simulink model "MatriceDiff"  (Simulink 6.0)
settings: Solver=ode45  StartTime=0  StopTime=17*t0  RelTol=1e-3
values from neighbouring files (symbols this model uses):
  b = S/Sm    (= 0.1)    [Constantes.m]    (also in ConstantesBck.m)
  beta = 0.95    [Constantes.m]    (also in ConstantesBck.m; ResCourV1.m = 1; ResCrV1.m = 1; ResEnerV1.m = 1)
  C = 1    [Constantes.m]    (also in ConstantesBck.m)
  gk = 36    [Constantes.m]    (also in ConstantesBck.m; sim_hh.m)
  gl = 0.3    [Constantes.m]    (also in ConstantesBck.m; sim_hh.m)
  gna = 120    [Constantes.m]    (also in ConstantesBck.m; sim_hh.m)
  h0 = 0.5961    [Constantes.m]    (also in ConstantesBck.m)
  m0 = 0.0529    [Constantes.m]    (also in ConstantesBck.m)
  mK = 0    [Constantes.m]    (also in ConstantesBck.m)
  mL = 0    [Constantes.m]    (also in ConstantesBck.m)
  mNa = 0    [Constantes.m]    (also in ConstantesBck.m)
  N = [6,8,5,5,7,1,2,6,9,1,1,9,4,8,8,7]    [Constantes.m]    (also in ConstantesBck.m; ImpedanceZtissus.m = 100; Ztissus.m = 100; charge.m = N(:,2))
  n0 = 0.3177    [Constantes.m]    (also in ConstantesBck.m)
  rapportIE = 10    [Constantes.m]
  Sm = 3.14e-2    (= 0.0314)    [Constantes.m]    (also in ConstantesBck.m = 0.000314)
  t0 = 2E-3    (= 0.002)    [Constantes.m]    (also in ConstantesBck.m = 0.001)
  Vk = -82    [Constantes.m]    (also in ConstantesBck.m)
  Vl = -59    [Constantes.m]    (also in ConstantesBck.m)
  Vna = 45    [Constantes.m]    (also in ConstantesBck.m)
  Vr = -70    [Constantes.m]    (also in ConstantesBck.m)
undefined symbols (not defined in the file or in its folder): ln
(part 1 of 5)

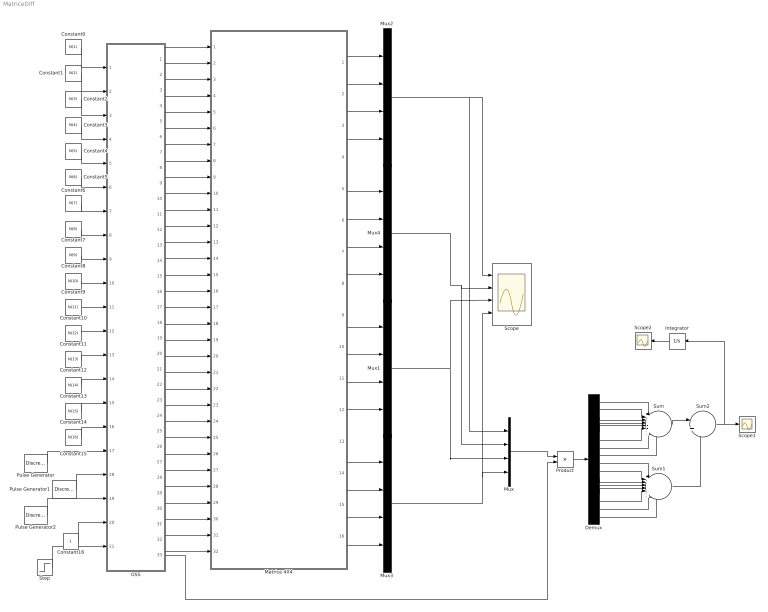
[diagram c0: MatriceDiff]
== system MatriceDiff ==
  Constant0 : Constant  Value=N(1)
  Constant1 : Constant  Value=N(2)
  Constant10 : Constant  Value=N(11)
  Constant11 : Constant  Value=N(12)
  Constant12 : Constant  Value=N(13)
  Constant13 : Constant  Value=N(14)
  Constant14 : Constant  Value=N(15)
  Constant15 : Constant  Value=N(16)
  Constant16 : Constant
  Constant2 : Constant  Value=N(3)
  Constant3 : Constant  Value=N(4)
  Constant4 : Constant  Value=N(5)
  Constant5 : Constant  Value=N(6)
  Constant6 : Constant  Value=N(7)
  Constant7 : Constant  Value=N(8)
  Constant8 : Constant  Value=N(9)
  Constant9 : Constant  Value=N(10)
  Demux : Demux  Outputs=16
  Integrator : Integrator  Orientation=left
  Matrice 4X4 : Subsystem
  Mux{,1..4} (5 alike) : Mux
  OSS : Stateflow chart
  Product : Product
  Pulse Generator : DiscretePulseGenerator  PulseType=Time based  Period=2*t0  PulseWidth=50  PhaseDelay=2*t0
  Pulse Generator1 : DiscretePulseGenerator  PulseType=Time based  Period=4*t0  PulseWidth=50  PhaseDelay=3*t0
  Pulse Generator2 : DiscretePulseGenerator  PulseType=Time based  Period=8*t0  PulseWidth=50  PhaseDelay=5*t0
  Scope : Scope  NumInputPorts=4
  Scope1 : Scope
  Scope2 : Scope
  Step : Step  Time=t0  SampleTime=0
  Sum : Sum  Inputs=|++++++++
  Sum1 : Sum  Inputs=|++++++++
  Sum2 : Sum  Inputs=|++
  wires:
  Matrice 4X4/13(Out12) -> Mux3/1
  Matrice 4X4/14(Out13) -> Mux3/2
  Matrice 4X4/15(Out14) -> Mux3/3
  Matrice 4X4/16(Out15) -> Mux3/4
  Constant14/1 -> OSS/15(u14)
  Constant13/1 -> OSS/14(u13)
  Constant12/1 -> OSS/13(u12)
  Constant11/1 -> OSS/12(u11)
  Constant10/1 -> OSS/11(u10)
  Constant9/1 -> OSS/10(u9)
  Constant8/1 -> OSS/9(u8)
  Constant7/1 -> OSS/8(u7)
  Constant6/1 -> OSS/7(u6)
  Constant5/1 -> OSS/6(u5)
  Constant4/1 -> OSS/5(u4)
  Constant3/1 -> OSS/4(u3)
  Constant2/1 -> OSS/3(u2)
  Constant1/1 -> OSS/2(u1)
  Constant0/1 -> OSS/1(u0)
  Constant15/1 -> OSS/16(u15)
  OSS/5(S2) -> Matrice 4X4/5(S2)
  OSS/6(Ref2) -> Matrice 4X4/6(Ref2)
  OSS/7(S3) -> Matrice 4X4/7(S3)
  OSS/8(Ref3) -> Matrice 4X4/8(Ref3)
  OSS/9(S4) -> Matrice 4X4/9(S4)
  OSS/10(Ref4) -> Matrice 4X4/10(Ref4)
  OSS/11(S5) -> Matrice 4X4/11(S5)
  OSS/12(Ref5) -> Matrice 4X4/12(Ref5)
  OSS/13(S6) -> Matrice 4X4/13(S6)
  OSS/14(Ref6) -> Matrice 4X4/14(Ref6)
  OSS/15(S7) -> Matrice 4X4/15(S7)
  OSS/16(Ref7) -> Matrice 4X4/16(Ref7)
  OSS/17(S8) -> Matrice 4X4/17(S8)
  OSS/18(Ref8) -> Matrice 4X4/18(Ref8)
  OSS/19(S9) -> Matrice 4X4/19(S9)
  OSS/20(Ref9) -> Matrice 4X4/20(Ref9)
  OSS/21(S10) -> Matrice 4X4/21(S10)
  OSS/22(Ref10) -> Matrice 4X4/22(Ref10)
  OSS/23(S11) -> Matrice 4X4/23(S11)
  OSS/24(Ref11) -> Matrice 4X4/24(Ref11)
  OSS/25(S12) -> Matrice 4X4/25(S12)
  OSS/26(Ref12) -> Matrice 4X4/26(Ref12)
  OSS/27(S13) -> Matrice 4X4/27(S13)
  OSS/28(Ref13) -> Matrice 4X4/28(Ref13)
  OSS/29(S14) -> Matrice 4X4/29(S14)
  OSS/30(Ref14) -> Matrice 4X4/30(Ref14)
  OSS/31(S15) -> Matrice 4X4/31(S15)
  OSS/32(Ref15) -> Matrice 4X4/32(Ref15)
  OSS/4(Ref1) -> Matrice 4X4/4(Ref1)
  OSS/3(S1) -> Matrice 4X4/3(S1)
  OSS/2(Ref0) -> Matrice 4X4/2(Ref0)
  OSS/1(S0) -> Matrice 4X4/1(S0)
  Pulse Generator/1 -> OSS/17(tc0)
  Pulse Generator2/1 -> OSS/19(tc2)
  Pulse Generator1/1 -> OSS/18(tc1)
  Mux3/1 -> Scope/4, Mux/4
  Matrice 4X4/9(Out8) -> Mux1/1
  Matrice 4X4/10(Out9) -> Mux1/2
  Matrice 4X4/12(Out11) -> Mux1/4
  Matrice 4X4/11(Out10) -> Mux1/3
  Matrice 4X4/5(Out4) -> Mux4/1
  Matrice 4X4/6(Out5) -> Mux4/2
  Matrice 4X4/7(Out6) -> Mux4/3
  Matrice 4X4/8(Out7) -> Mux4/4
  Matrice 4X4/1(Out0) -> Mux2/1
  Matrice 4X4/2(Out1) -> Mux2/2
  Matrice 4X4/4(Out3) -> Mux2/4
  Matrice 4X4/3(Out2) -> Mux2/3
  Mux1/1 -> Scope/3, Mux/3
  Mux4/1 -> Scope/2, Mux/2
  Mux2/1 -> Scope/1, Mux/1
  Constant16/1 -> OSS/20(dyn)
  OSS/33(MatCourant) -> Product/2
  Mux/1 -> Product/1
  Product/1 -> Demux/1
  Demux/1 -> Sum/1
  Demux/2 -> Sum/2
  Demux/3 -> Sum/3
  Demux/4 -> Sum/4
  Demux/5 -> Sum/5
  Demux/6 -> Sum/6
  Demux/7 -> Sum/7
  Demux/8 -> Sum/8
  Demux/9 -> Sum1/1
  Demux/10 -> Sum1/2
  Demux/11 -> Sum1/3
  Demux/12 -> Sum1/4
  Demux/13 -> Sum1/5
  Demux/14 -> Sum1/6
  Demux/15 -> Sum1/7
  Demux/16 -> Sum1/8
  Sum/1 -> Sum2/1
  Sum1/1 -> Sum2/2
  Sum2/1 -> Scope1/1, Integrator/1
  Integrator/1 -> Scope2/1
  Step/1 -> OSS/21(rst)

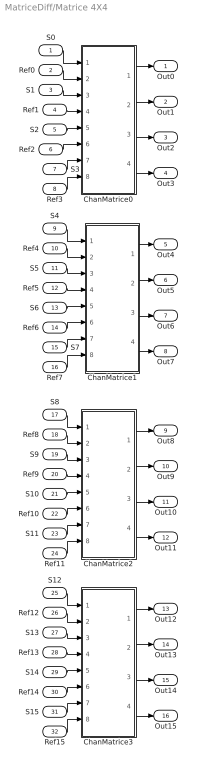
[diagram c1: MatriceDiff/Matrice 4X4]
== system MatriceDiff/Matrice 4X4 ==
  S0 : Inport  Port=1  LatchInput=off
  Ref0 : Inport  Port=2  LatchInput=off
  S1 : Inport  Port=3  LatchInput=off
  Ref1 : Inport  Port=4  LatchInput=off
  S2 : Inport  Port=5  LatchInput=off
  Ref2 : Inport  Port=6  LatchInput=off
  S3 : Inport  Port=7  LatchInput=off
  Ref3 : Inport  Port=8  LatchInput=off
  S4 : Inport  Port=9  LatchInput=off
  Ref4 : Inport  Port=10  LatchInput=off
  S5 : Inport  Port=11  LatchInput=off
  Ref5 : Inport  Port=12  LatchInput=off
  S6 : Inport  Port=13  LatchInput=off
  Ref6 : Inport  Port=14  LatchInput=off
  S7 : Inport  Port=15  LatchInput=off
  Ref7 : Inport  Port=16  LatchInput=off
  S8 : Inport  Port=17  LatchInput=off
  Ref8 : Inport  Port=18  LatchInput=off
  S9 : Inport  Port=19  LatchInput=off
  Ref9 : Inport  Port=20  LatchInput=off
  S10 : Inport  Port=21  LatchInput=off
  Ref10 : Inport  Port=22  LatchInput=off
  S11 : Inport  Port=23  LatchInput=off
  Ref11 : Inport  Port=24  LatchInput=off
  S12 : Inport  Port=25  LatchInput=off
  Ref12 : Inport  Port=26  LatchInput=off
  S13 : Inport  Port=27  LatchInput=off
  Ref13 : Inport  Port=28  LatchInput=off
  S14 : Inport  Port=29  LatchInput=off
  Ref14 : Inport  Port=30  LatchInput=off
  S15 : Inport  Port=31  LatchInput=off
  Ref15 : Inport  Port=32  LatchInput=off
  ChanMatrice0 : Subsystem
  ChanMatrice1 : Subsystem
  ChanMatrice2 : Subsystem
  ChanMatrice3 : Subsystem
  Out0 : Outport
  Out1 : Outport  Port=2
  Out2 : Outport  Port=3
  Out3 : Outport  Port=4
  Out4 : Outport  Port=5
  Out5 : Outport  Port=6
  Out6 : Outport  Port=7
  Out7 : Outport  Port=8
  Out8 : Outport  Port=9
  Out9 : Outport  Port=10
  Out10 : Outport  Port=11
  Out11 : Outport  Port=12
  Out12 : Outport  Port=13
  Out13 : Outport  Port=14
  Out14 : Outport  Port=15
  Out15 : Outport  Port=16
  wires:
  S0/1 -> ChanMatrice0/1(S0)
  ChanMatrice0/1(Out0) -> Out0/1
  Ref0/1 -> ChanMatrice0/2(Ref0)
  S1/1 -> ChanMatrice0/3(S1)
  ChanMatrice0/2(Out1) -> Out1/1
  ChanMatrice0/3(Out2) -> Out2/1
  ChanMatrice0/4(Out3) -> Out3/1
  ChanMatrice1/1(Out0) -> Out4/1
  ChanMatrice1/2(Out1) -> Out5/1
  ChanMatrice1/3(Out2) -> Out6/1
  ChanMatrice1/4(Out3) -> Out7/1
  ChanMatrice2/1(Out0) -> Out8/1
  ChanMatrice2/2(Out1) -> Out9/1
  ChanMatrice2/3(Out2) -> Out10/1
  ChanMatrice2/4(Out3) -> Out11/1
  ChanMatrice3/1(Out0) -> Out12/1
  ChanMatrice3/2(Out1) -> Out13/1
  ChanMatrice3/3(Out2) -> Out14/1
  ChanMatrice3/4(Out3) -> Out15/1
  S2/1 -> ChanMatrice0/5(S2)
  S3/1 -> ChanMatrice0/7(S3)
  S4/1 -> ChanMatrice1/1(S0)
  S5/1 -> ChanMatrice1/3(S1)
  S6/1 -> ChanMatrice1/5(S2)
  S7/1 -> ChanMatrice1/7(S3)
  S12/1 -> ChanMatrice3/1(S0)
  S13/1 -> ChanMatrice3/3(S1)
  S14/1 -> ChanMatrice3/5(S2)
  S15/1 -> ChanMatrice3/7(S3)
  S8/1 -> ChanMatrice2/1(S0)
  S9/1 -> ChanMatrice2/3(S1)
  S10/1 -> ChanMatrice2/5(S2)
  S11/1 -> ChanMatrice2/7(S3)
  Ref1/1 -> ChanMatrice0/4(Ref1)
  Ref2/1 -> ChanMatrice0/6(Ref2)
  Ref3/1 -> ChanMatrice0/8(Ref3)
  Ref4/1 -> ChanMatrice1/2(Ref0)
  Ref5/1 -> ChanMatrice1/4(Ref1)
  Ref6/1 -> ChanMatrice1/6(Ref2)
  Ref7/1 -> ChanMatrice1/8(Ref3)
  Ref8/1 -> ChanMatrice2/2(Ref0)
  Ref9/1 -> ChanMatrice2/4(Ref1)
  Ref10/1 -> ChanMatrice2/6(Ref2)
  Ref11/1 -> ChanMatrice2/8(Ref3)
  Ref12/1 -> ChanMatrice3/2(Ref0)
  Ref13/1 -> ChanMatrice3/4(Ref1)
  Ref14/1 -> ChanMatrice3/6(Ref2)
  Ref15/1 -> ChanMatrice3/8(Ref3)

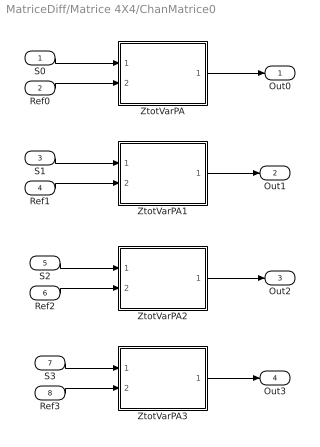
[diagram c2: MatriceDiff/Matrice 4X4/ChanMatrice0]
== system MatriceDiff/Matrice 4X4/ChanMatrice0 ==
  S0 : Inport  Port=1  LatchInput=off
  Ref0 : Inport  Port=2  LatchInput=off
  S1 : Inport  Port=3  LatchInput=off
  Ref1 : Inport  Port=4  LatchInput=off
  S2 : Inport  Port=5  LatchInput=off
  Ref2 : Inport  Port=6  LatchInput=off
  S3 : Inport  Port=7  LatchInput=off
  Ref3 : Inport  Port=8  LatchInput=off
  ZtotVarPA : Subsystem
  ZtotVarPA1 : Subsystem
  ZtotVarPA2 : Subsystem
  ZtotVarPA3 : Subsystem
  Out0 : Outport
  Out1 : Outport  Port=2
  Out2 : Outport  Port=3
  Out3 : Outport  Port=4
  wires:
  S0/1 -> ZtotVarPA/1(InZtot)
  Ref0/1 -> ZtotVarPA/2(InVref)
  ZtotVarPA/1(OutZtot) -> Out0/1
  ZtotVarPA1/1(OutZtot) -> Out1/1
  ZtotVarPA2/1(OutZtot) -> Out2/1
  ZtotVarPA3/1(OutZtot) -> Out3/1
  S1/1 -> ZtotVarPA1/1(InZtot)
  Ref1/1 -> ZtotVarPA1/2(InVref)
  S2/1 -> ZtotVarPA2/1(InZtot)
  Ref2/1 -> ZtotVarPA2/2(InVref)
  S3/1 -> ZtotVarPA3/1(InZtot)
  Ref3/1 -> ZtotVarPA3/2(InVref)

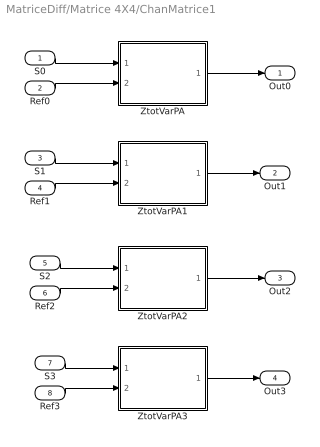
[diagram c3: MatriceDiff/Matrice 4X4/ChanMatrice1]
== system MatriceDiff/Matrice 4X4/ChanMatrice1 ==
  S0 : Inport  Port=1  LatchInput=off
  Ref0 : Inport  Port=2  LatchInput=off
  S1 : Inport  Port=3  LatchInput=off
  Ref1 : Inport  Port=4  LatchInput=off
  S2 : Inport  Port=5  LatchInput=off
  Ref2 : Inport  Port=6  LatchInput=off
  S3 : Inport  Port=7  LatchInput=off
  Ref3 : Inport  Port=8  LatchInput=off
  ZtotVarPA : Subsystem
  ZtotVarPA1 : Subsystem
  ZtotVarPA2 : Subsystem
  ZtotVarPA3 : Subsystem
  Out0 : Outport
  Out1 : Outport  Port=2
  Out2 : Outport  Port=3
  Out3 : Outport  Port=4
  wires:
  S0/1 -> ZtotVarPA/1(InZtot)
  Ref0/1 -> ZtotVarPA/2(InVref)
  ZtotVarPA/1(OutZtot) -> Out0/1
  ZtotVarPA1/1(OutZtot) -> Out1/1
  ZtotVarPA2/1(OutZtot) -> Out2/1
  ZtotVarPA3/1(OutZtot) -> Out3/1
  S1/1 -> ZtotVarPA1/1(InZtot)
  Ref1/1 -> ZtotVarPA1/2(InVref)
  S2/1 -> ZtotVarPA2/1(InZtot)
  Ref2/1 -> ZtotVarPA2/2(InVref)
  S3/1 -> ZtotVarPA3/1(InZtot)
  Ref3/1 -> ZtotVarPA3/2(InVref)

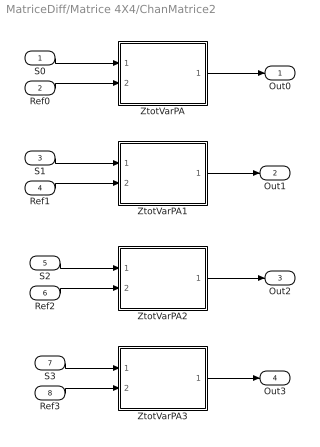
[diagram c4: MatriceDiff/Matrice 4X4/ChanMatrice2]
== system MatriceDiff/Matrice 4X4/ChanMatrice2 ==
  S0 : Inport  Port=1  LatchInput=off
  Ref0 : Inport  Port=2  LatchInput=off
  S1 : Inport  Port=3  LatchInput=off
  Ref1 : Inport  Port=4  LatchInput=off
  S2 : Inport  Port=5  LatchInput=off
  Ref2 : Inport  Port=6  LatchInput=off
  S3 : Inport  Port=7  LatchInput=off
  Ref3 : Inport  Port=8  LatchInput=off
  ZtotVarPA : Subsystem
  ZtotVarPA1 : Subsystem
  ZtotVarPA2 : Subsystem
  ZtotVarPA3 : Subsystem
  Out0 : Outport
  Out1 : Outport  Port=2
  Out2 : Outport  Port=3
  Out3 : Outport  Port=4
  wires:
  S0/1 -> ZtotVarPA/1(InZtot)
  Ref0/1 -> ZtotVarPA/2(InVref)
  ZtotVarPA/1(OutZtot) -> Out0/1
  ZtotVarPA1/1(OutZtot) -> Out1/1
  ZtotVarPA2/1(OutZtot) -> Out2/1
  ZtotVarPA3/1(OutZtot) -> Out3/1
  S1/1 -> ZtotVarPA1/1(InZtot)
  Ref1/1 -> ZtotVarPA1/2(InVref)
  S2/1 -> ZtotVarPA2/1(InZtot)
  Ref2/1 -> ZtotVarPA2/2(InVref)
  S3/1 -> ZtotVarPA3/1(InZtot)
  Ref3/1 -> ZtotVarPA3/2(InVref)

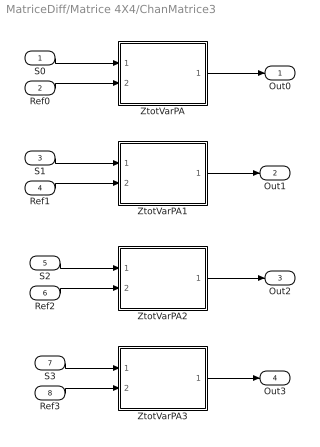
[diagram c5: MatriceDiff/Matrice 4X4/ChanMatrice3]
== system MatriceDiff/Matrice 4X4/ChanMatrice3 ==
  S0 : Inport  Port=1  LatchInput=off
  Ref0 : Inport  Port=2  LatchInput=off
  S1 : Inport  Port=3  LatchInput=off
  Ref1 : Inport  Port=4  LatchInput=off
  S2 : Inport  Port=5  LatchInput=off
  Ref2 : Inport  Port=6  LatchInput=off
  S3 : Inport  Port=7  LatchInput=off
  Ref3 : Inport  Port=8  LatchInput=off
  ZtotVarPA : Subsystem
  ZtotVarPA1 : Subsystem
  ZtotVarPA2 : Subsystem
  ZtotVarPA3 : Subsystem
  Out0 : Outport
  Out1 : Outport  Port=2
  Out2 : Outport  Port=3
  Out3 : Outport  Port=4
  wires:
  S0/1 -> ZtotVarPA/1(InZtot)
  Ref0/1 -> ZtotVarPA/2(InVref)
  ZtotVarPA/1(OutZtot) -> Out0/1
  ZtotVarPA1/1(OutZtot) -> Out1/1
  ZtotVarPA2/1(OutZtot) -> Out2/1
  ZtotVarPA3/1(OutZtot) -> Out3/1
  S1/1 -> ZtotVarPA1/1(InZtot)
  Ref1/1 -> ZtotVarPA1/2(InVref)
  S2/1 -> ZtotVarPA2/1(InZtot)
  Ref2/1 -> ZtotVarPA2/2(InVref)
  S3/1 -> ZtotVarPA3/1(InZtot)
  Ref3/1 -> ZtotVarPA3/2(InVref)

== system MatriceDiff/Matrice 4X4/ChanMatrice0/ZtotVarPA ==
  InZtot : Inport  Port=1  LatchInput=off
  InVref : Inport  Port=2  LatchInput=off
  Gain : Gain
  Sum : Sum  Inputs=|++
  ZTissusVar : Subsystem
  ZietVar : Subsystem
  OutZtot : Outport
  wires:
  ZietVar/1(OutZiet) -> Gain/1
  ZTissusVar/1(Vout) -> Sum/1
  InZtot/1 -> ZTissusVar/1(IStim), ZietVar/1(InZiet)
  Gain/1 -> Sum/2
  Sum/1 -> OutZtot/1
  InVref/1 -> ZTissusVar/2(Vref)

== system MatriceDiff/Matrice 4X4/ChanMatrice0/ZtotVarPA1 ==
  InZtot : Inport  Port=1  LatchInput=off
  InVref : Inport  Port=2  LatchInput=off
  Gain : Gain
  Sum : Sum  Inputs=|++
  ZTissusVar : Subsystem
  ZietVar : Subsystem
  OutZtot : Outport
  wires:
  ZietVar/1(OutZiet) -> Gain/1
  ZTissusVar/1(Vout) -> Sum/1
  InZtot/1 -> ZTissusVar/1(IStim), ZietVar/1(InZiet)
  Gain/1 -> Sum/2
  Sum/1 -> OutZtot/1
  InVref/1 -> ZTissusVar/2(Vref)

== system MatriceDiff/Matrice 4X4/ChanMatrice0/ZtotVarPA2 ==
  InZtot : Inport  Port=1  LatchInput=off
  InVref : Inport  Port=2  LatchInput=off
  Gain : Gain
  Sum : Sum  Inputs=|++
  ZTissusVar : Subsystem
  ZietVar : Subsystem
  OutZtot : Outport
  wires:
  ZietVar/1(OutZiet) -> Gain/1
  ZTissusVar/1(Vout) -> Sum/1
  InZtot/1 -> ZTissusVar/1(IStim), ZietVar/1(InZiet)
  Gain/1 -> Sum/2
  Sum/1 -> OutZtot/1
  InVref/1 -> ZTissusVar/2(Vref)

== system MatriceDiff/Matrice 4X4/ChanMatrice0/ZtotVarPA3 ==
  InZtot : Inport  Port=1  LatchInput=off
  InVref : Inport  Port=2  LatchInput=off
  Gain : Gain
  Sum : Sum  Inputs=|++
  ZTissusVar : Subsystem
  ZietVar : Subsystem
  OutZtot : Outport
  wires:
  ZietVar/1(OutZiet) -> Gain/1
  ZTissusVar/1(Vout) -> Sum/1
  InZtot/1 -> ZTissusVar/1(IStim), ZietVar/1(InZiet)
  Gain/1 -> Sum/2
  Sum/1 -> OutZtot/1
  InVref/1 -> ZTissusVar/2(Vref)

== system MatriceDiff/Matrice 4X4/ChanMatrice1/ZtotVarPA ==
  InZtot : Inport  Port=1  LatchInput=off
  InVref : Inport  Port=2  LatchInput=off
  Gain : Gain
  Sum : Sum  Inputs=|++
  ZTissusVar : Subsystem
  ZietVar : Subsystem
  OutZtot : Outport
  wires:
  ZietVar/1(OutZiet) -> Gain/1
  ZTissusVar/1(Vout) -> Sum/1
  InZtot/1 -> ZTissusVar/1(IStim), ZietVar/1(InZiet)
  Gain/1 -> Sum/2
  Sum/1 -> OutZtot/1
  InVref/1 -> ZTissusVar/2(Vref)

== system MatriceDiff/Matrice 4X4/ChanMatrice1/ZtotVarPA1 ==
  InZtot : Inport  Port=1  LatchInput=off
  InVref : Inport  Port=2  LatchInput=off
  Gain : Gain
  Sum : Sum  Inputs=|++
  ZTissusVar : Subsystem
  ZietVar : Subsystem
  OutZtot : Outport
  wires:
  ZietVar/1(OutZiet) -> Gain/1
  ZTissusVar/1(Vout) -> Sum/1
  InZtot/1 -> ZTissusVar/1(IStim), ZietVar/1(InZiet)
  Gain/1 -> Sum/2
  Sum/1 -> OutZtot/1
  InVref/1 -> ZTissusVar/2(Vref)

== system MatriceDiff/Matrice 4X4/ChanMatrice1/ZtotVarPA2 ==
  InZtot : Inport  Port=1  LatchInput=off
  InVref : Inport  Port=2  LatchInput=off
  Gain : Gain
  Sum : Sum  Inputs=|++
  ZTissusVar : Subsystem
  ZietVar : Subsystem
  OutZtot : Outport
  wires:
  ZietVar/1(OutZiet) -> Gain/1
  ZTissusVar/1(Vout) -> Sum/1
  InZtot/1 -> ZTissusVar/1(IStim), ZietVar/1(InZiet)
  Gain/1 -> Sum/2
  Sum/1 -> OutZtot/1
  InVref/1 -> ZTissusVar/2(Vref)

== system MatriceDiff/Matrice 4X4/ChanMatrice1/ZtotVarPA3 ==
  InZtot : Inport  Port=1  LatchInput=off
  InVref : Inport  Port=2  LatchInput=off
  Gain : Gain
  Sum : Sum  Inputs=|++
  ZTissusVar : Subsystem
  ZietVar : Subsystem
  OutZtot : Outport
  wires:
  ZietVar/1(OutZiet) -> Gain/1
  ZTissusVar/1(Vout) -> Sum/1
  InZtot/1 -> ZTissusVar/1(IStim), ZietVar/1(InZiet)
  Gain/1 -> Sum/2
  Sum/1 -> OutZtot/1
  InVref/1 -> ZTissusVar/2(Vref)

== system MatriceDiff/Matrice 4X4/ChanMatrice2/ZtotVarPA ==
  InZtot : Inport  Port=1  LatchInput=off
  InVref : Inport  Port=2  LatchInput=off
  Gain : Gain
  Sum : Sum  Inputs=|++
  ZTissusVar : Subsystem
  ZietVar : Subsystem
  OutZtot : Outport
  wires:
  ZietVar/1(OutZiet) -> Gain/1
  ZTissusVar/1(Vout) -> Sum/1
  InZtot/1 -> ZTissusVar/1(IStim), ZietVar/1(InZiet)
  Gain/1 -> Sum/2
  Sum/1 -> OutZtot/1
  InVref/1 -> ZTissusVar/2(Vref)

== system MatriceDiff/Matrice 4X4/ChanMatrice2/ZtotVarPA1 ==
  InZtot : Inport  Port=1  LatchInput=off
  InVref : Inport  Port=2  LatchInput=off
  Gain : Gain
  Sum : Sum  Inputs=|++
  ZTissusVar : Subsystem
  ZietVar : Subsystem
  OutZtot : Outport
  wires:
  ZietVar/1(OutZiet) -> Gain/1
  ZTissusVar/1(Vout) -> Sum/1
  InZtot/1 -> ZTissusVar/1(IStim), ZietVar/1(InZiet)
  Gain/1 -> Sum/2
  Sum/1 -> OutZtot/1
  InVref/1 -> ZTissusVar/2(Vref)

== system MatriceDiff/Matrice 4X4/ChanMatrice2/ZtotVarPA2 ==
  InZtot : Inport  Port=1  LatchInput=off
  InVref : Inport  Port=2  LatchInput=off
  Gain : Gain
  Sum : Sum  Inputs=|++
  ZTissusVar : Subsystem
  ZietVar : Subsystem
  OutZtot : Outport
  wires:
  ZietVar/1(OutZiet) -> Gain/1
  ZTissusVar/1(Vout) -> Sum/1
  InZtot/1 -> ZTissusVar/1(IStim), ZietVar/1(InZiet)
  Gain/1 -> Sum/2
  Sum/1 -> OutZtot/1
  InVref/1 -> ZTissusVar/2(Vref)

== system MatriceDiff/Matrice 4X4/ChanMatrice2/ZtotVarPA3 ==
  InZtot : Inport  Port=1  LatchInput=off
  InVref : Inport  Port=2  LatchInput=off
  Gain : Gain
  Sum : Sum  Inputs=|++
  ZTissusVar : Subsystem
  ZietVar : Subsystem
  OutZtot : Outport
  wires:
  ZietVar/1(OutZiet) -> Gain/1
  ZTissusVar/1(Vout) -> Sum/1
  InZtot/1 -> ZTissusVar/1(IStim), ZietVar/1(InZiet)
  Gain/1 -> Sum/2
  Sum/1 -> OutZtot/1
  InVref/1 -> ZTissusVar/2(Vref)

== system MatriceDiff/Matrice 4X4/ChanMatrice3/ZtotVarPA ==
  InZtot : Inport  Port=1  LatchInput=off
  InVref : Inport  Port=2  LatchInput=off
  Gain : Gain
  Sum : Sum  Inputs=|++
  ZTissusVar : Subsystem
  ZietVar : Subsystem
  OutZtot : Outport
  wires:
  ZietVar/1(OutZiet) -> Gain/1
  ZTissusVar/1(Vout) -> Sum/1
  InZtot/1 -> ZTissusVar/1(IStim), ZietVar/1(InZiet)
  Gain/1 -> Sum/2
  Sum/1 -> OutZtot/1
  InVref/1 -> ZTissusVar/2(Vref)

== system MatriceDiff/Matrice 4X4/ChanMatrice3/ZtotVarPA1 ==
  InZtot : Inport  Port=1  LatchInput=off
  InVref : Inport  Port=2  LatchInput=off
  Gain : Gain
  Sum : Sum  Inputs=|++
  ZTissusVar : Subsystem
  ZietVar : Subsystem
  OutZtot : Outport
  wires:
  ZietVar/1(OutZiet) -> Gain/1
  ZTissusVar/1(Vout) -> Sum/1
  InZtot/1 -> ZTissusVar/1(IStim), ZietVar/1(InZiet)
  Gain/1 -> Sum/2
  Sum/1 -> OutZtot/1
  InVref/1 -> ZTissusVar/2(Vref)

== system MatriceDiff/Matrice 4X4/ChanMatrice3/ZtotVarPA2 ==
  InZtot : Inport  Port=1  LatchInput=off
  InVref : Inport  Port=2  LatchInput=off
  Gain : Gain
  Sum : Sum  Inputs=|++
  ZTissusVar : Subsystem
  ZietVar : Subsystem
  OutZtot : Outport
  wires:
  ZietVar/1(OutZiet) -> Gain/1
  ZTissusVar/1(Vout) -> Sum/1
  InZtot/1 -> ZTissusVar/1(IStim), ZietVar/1(InZiet)
  Gain/1 -> Sum/2
  Sum/1 -> OutZtot/1
  InVref/1 -> ZTissusVar/2(Vref)

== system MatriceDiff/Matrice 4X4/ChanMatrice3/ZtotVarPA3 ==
  InZtot : Inport  Port=1  LatchInput=off
  InVref : Inport  Port=2  LatchInput=off
  Gain : Gain
  Sum : Sum  Inputs=|++
  ZTissusVar : Subsystem
  ZietVar : Subsystem
  OutZtot : Outport
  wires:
  ZietVar/1(OutZiet) -> Gain/1
  ZTissusVar/1(Vout) -> Sum/1
  InZtot/1 -> ZTissusVar/1(IStim), ZietVar/1(InZiet)
  Gain/1 -> Sum/2
  Sum/1 -> OutZtot/1
  InVref/1 -> ZTissusVar/2(Vref)

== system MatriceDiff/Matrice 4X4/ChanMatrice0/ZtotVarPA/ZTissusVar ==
  IStim : Inport  Orientation=left  Port=1  LatchInput=off
  Vref : Inport  Port=2  LatchInput=off
  Constant : Constant
  Contrôleur : Stateflow chart  Orientation=left
  Divide : Product  Inputs=*/  OutScaling=2^-10
  Divide1 : Product  Inputs=*/  OutScaling=2^-10
  Divide2 : Product  Inputs=*/  OutScaling=2^-10
  Rext1 : Fcn  Expr=u*(1.6342*((abs(u)*1E6)^0.1267))*1E3
  Sum1 : Sum  Inputs=|++
  ZTissusInt : Subsystem
  Vout : Outport  Orientation=left
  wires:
  Constant/1 -> Divide/1, Divide1/1, Divide2/1
  ZTissusInt/1(Vout) -> Divide/2
  Rext1/1 -> Divide1/2
  Divide/1 -> Sum1/1
  Divide1/1 -> Sum1/2
  Sum1/1 -> Divide2/2
  Vref/1 -> ZTissusInt/2(VRefIn)
  Divide2/1 -> Contrôleur/2(calc)
  Contrôleur/2(temp) -> Rext1/1, ZTissusInt/1(InStim)
  IStim/1 -> Contrôleur/1(u)
  Contrôleur/1(y) -> Vout/1

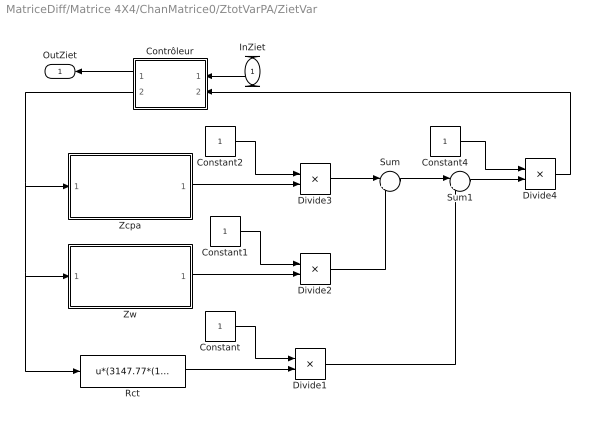
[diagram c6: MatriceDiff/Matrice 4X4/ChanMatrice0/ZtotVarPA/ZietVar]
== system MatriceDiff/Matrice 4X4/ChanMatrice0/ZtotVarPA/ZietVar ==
  InZiet : Inport  Orientation=left  Port=1  LatchInput=off
  Constant{,1..2,4} (4 alike) : Constant
  Contrôleur : Stateflow chart  Orientation=left
  Divide{1..4} (4 alike) : Product  Inputs=*/  OutScaling=2^-10
  Rct : Fcn  Expr=u*(3147.77*(1/((1E6*abs(u))^0.7199)))*1000
  Sum : Sum  Inputs=|++
  Sum1 : Sum  Inputs=|++
  Zcpa : Subsystem
  Zw : Subsystem
  OutZiet : Outport  Orientation=left
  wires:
  Constant/1 -> Divide1/1
  Constant1/1 -> Divide2/1
  Constant2/1 -> Divide3/1
  Zcpa/1(OutZcpa) -> Divide3/2
  Zw/1(OutZw) -> Divide2/2
  Rct/1 -> Divide1/2
  Divide3/1 -> Sum/1
  Constant4/1 -> Divide4/1
  Divide2/1 -> Sum/2
  Sum/1 -> Sum1/1
  Divide1/1 -> Sum1/2
  Sum1/1 -> Divide4/2
  Contrôleur/2(temp) -> Rct/1, Zw/1(InZw), Zcpa/1(InZcpa)
  InZiet/1 -> Contrôleur/1(u)
  Contrôleur/1(y) -> OutZiet/1
  Divide4/1 -> Contrôleur/2(calc)

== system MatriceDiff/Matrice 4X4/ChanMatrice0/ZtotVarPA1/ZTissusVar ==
  IStim : Inport  Orientation=left  Port=1  LatchInput=off
  Vref : Inport  Port=2  LatchInput=off
  Constant : Constant
  Contrôleur : Stateflow chart  Orientation=left
  Divide : Product  Inputs=*/  OutScaling=2^-10
  Divide1 : Product  Inputs=*/  OutScaling=2^-10
  Divide2 : Product  Inputs=*/  OutScaling=2^-10
  Rext1 : Fcn  Expr=u*(1.6342*((abs(u)*1E6)^0.1267))*1E3
  Sum1 : Sum  Inputs=|++
  ZTissusInt : Subsystem
  Vout : Outport  Orientation=left
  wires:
  Constant/1 -> Divide/1, Divide1/1, Divide2/1
  ZTissusInt/1(Vout) -> Divide/2
  Rext1/1 -> Divide1/2
  Divide/1 -> Sum1/1
  Divide1/1 -> Sum1/2
  Sum1/1 -> Divide2/2
  Vref/1 -> ZTissusInt/2(VRefIn)
  Divide2/1 -> Contrôleur/2(calc)
  Contrôleur/2(temp) -> Rext1/1, ZTissusInt/1(InStim)
  IStim/1 -> Contrôleur/1(u)
  Contrôleur/1(y) -> Vout/1

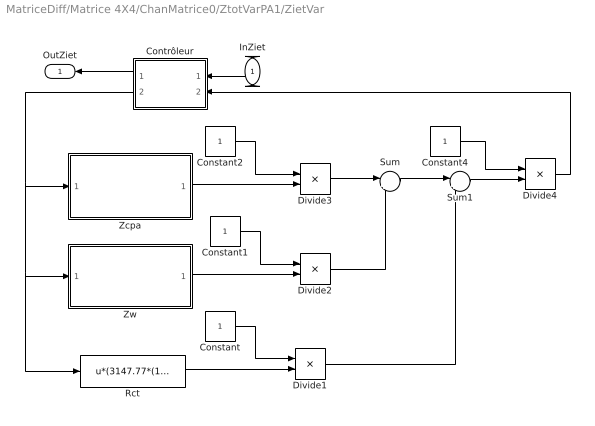
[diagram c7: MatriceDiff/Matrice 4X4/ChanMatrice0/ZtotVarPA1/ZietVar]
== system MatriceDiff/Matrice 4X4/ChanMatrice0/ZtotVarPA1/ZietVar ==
  InZiet : Inport  Orientation=left  Port=1  LatchInput=off
  Constant{,1..2,4} (4 alike) : Constant
  Contrôleur : Stateflow chart  Orientation=left
  Divide{1..4} (4 alike) : Product  Inputs=*/  OutScaling=2^-10
  Rct : Fcn  Expr=u*(3147.77*(1/((1E6*abs(u))^0.7199)))*1000
  Sum : Sum  Inputs=|++
  Sum1 : Sum  Inputs=|++
  Zcpa : Subsystem
  Zw : Subsystem
  OutZiet : Outport  Orientation=left
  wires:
  Constant/1 -> Divide1/1
  Constant1/1 -> Divide2/1
  Constant2/1 -> Divide3/1
  Zcpa/1(OutZcpa) -> Divide3/2
  Zw/1(OutZw) -> Divide2/2
  Rct/1 -> Divide1/2
  Divide3/1 -> Sum/1
  Constant4/1 -> Divide4/1
  Divide2/1 -> Sum/2
  Sum/1 -> Sum1/1
  Divide1/1 -> Sum1/2
  Sum1/1 -> Divide4/2
  Contrôleur/2(temp) -> Rct/1, Zw/1(InZw), Zcpa/1(InZcpa)
  InZiet/1 -> Contrôleur/1(u)
  Contrôleur/1(y) -> OutZiet/1
  Divide4/1 -> Contrôleur/2(calc)

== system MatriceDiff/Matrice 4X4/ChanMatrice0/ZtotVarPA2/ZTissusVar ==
  IStim : Inport  Orientation=left  Port=1  LatchInput=off
  Vref : Inport  Port=2  LatchInput=off
  Constant : Constant
  Contrôleur : Stateflow chart  Orientation=left
  Divide : Product  Inputs=*/  OutScaling=2^-10
  Divide1 : Product  Inputs=*/  OutScaling=2^-10
  Divide2 : Product  Inputs=*/  OutScaling=2^-10
  Rext1 : Fcn  Expr=u*(1.6342*((abs(u)*1E6)^0.1267))*1E3
  Sum1 : Sum  Inputs=|++
  ZTissusInt : Subsystem
  Vout : Outport  Orientation=left
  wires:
  Constant/1 -> Divide/1, Divide1/1, Divide2/1
  ZTissusInt/1(Vout) -> Divide/2
  Rext1/1 -> Divide1/2
  Divide/1 -> Sum1/1
  Divide1/1 -> Sum1/2
  Sum1/1 -> Divide2/2
  Vref/1 -> ZTissusInt/2(VRefIn)
  Divide2/1 -> Contrôleur/2(calc)
  Contrôleur/2(temp) -> Rext1/1, ZTissusInt/1(InStim)
  IStim/1 -> Contrôleur/1(u)
  Contrôleur/1(y) -> Vout/1

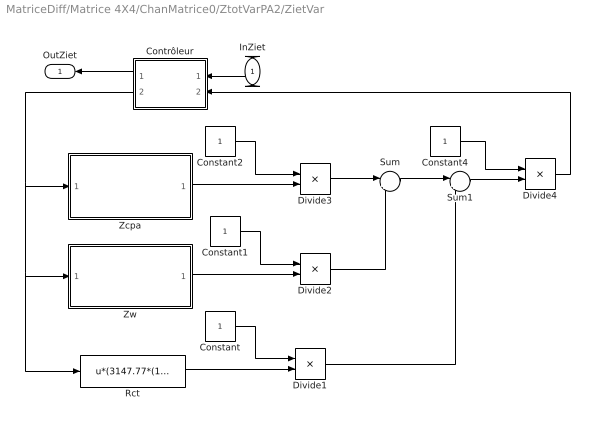
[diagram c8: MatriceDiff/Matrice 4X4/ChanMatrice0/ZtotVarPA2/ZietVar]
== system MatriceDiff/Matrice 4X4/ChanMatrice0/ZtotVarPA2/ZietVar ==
  InZiet : Inport  Orientation=left  Port=1  LatchInput=off
  Constant{,1..2,4} (4 alike) : Constant
  Contrôleur : Stateflow chart  Orientation=left
  Divide{1..4} (4 alike) : Product  Inputs=*/  OutScaling=2^-10
  Rct : Fcn  Expr=u*(3147.77*(1/((1E6*abs(u))^0.7199)))*1000
  Sum : Sum  Inputs=|++
  Sum1 : Sum  Inputs=|++
  Zcpa : Subsystem
  Zw : Subsystem
  OutZiet : Outport  Orientation=left
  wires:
  Constant/1 -> Divide1/1
  Constant1/1 -> Divide2/1
  Constant2/1 -> Divide3/1
  Zcpa/1(OutZcpa) -> Divide3/2
  Zw/1(OutZw) -> Divide2/2
  Rct/1 -> Divide1/2
  Divide3/1 -> Sum/1
  Constant4/1 -> Divide4/1
  Divide2/1 -> Sum/2
  Sum/1 -> Sum1/1
  Divide1/1 -> Sum1/2
  Sum1/1 -> Divide4/2
  Contrôleur/2(temp) -> Rct/1, Zw/1(InZw), Zcpa/1(InZcpa)
  InZiet/1 -> Contrôleur/1(u)
  Contrôleur/1(y) -> OutZiet/1
  Divide4/1 -> Contrôleur/2(calc)

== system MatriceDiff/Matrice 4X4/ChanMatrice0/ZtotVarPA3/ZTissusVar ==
  IStim : Inport  Orientation=left  Port=1  LatchInput=off
  Vref : Inport  Port=2  LatchInput=off
  Constant : Constant
  Contrôleur : Stateflow chart  Orientation=left
  Divide : Product  Inputs=*/  OutScaling=2^-10
  Divide1 : Product  Inputs=*/  OutScaling=2^-10
  Divide2 : Product  Inputs=*/  OutScaling=2^-10
  Rext1 : Fcn  Expr=u*(1.6342*((abs(u)*1E6)^0.1267))*1E3
  Sum1 : Sum  Inputs=|++
  ZTissusInt : Subsystem
  Vout : Outport  Orientation=left
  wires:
  Constant/1 -> Divide/1, Divide1/1, Divide2/1
  ZTissusInt/1(Vout) -> Divide/2
  Rext1/1 -> Divide1/2
  Divide/1 -> Sum1/1
  Divide1/1 -> Sum1/2
  Sum1/1 -> Divide2/2
  Vref/1 -> ZTissusInt/2(VRefIn)
  Divide2/1 -> Contrôleur/2(calc)
  Contrôleur/2(temp) -> Rext1/1, ZTissusInt/1(InStim)
  IStim/1 -> Contrôleur/1(u)
  Contrôleur/1(y) -> Vout/1

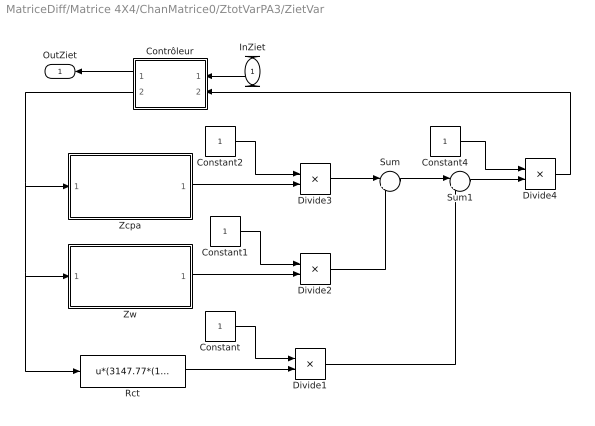
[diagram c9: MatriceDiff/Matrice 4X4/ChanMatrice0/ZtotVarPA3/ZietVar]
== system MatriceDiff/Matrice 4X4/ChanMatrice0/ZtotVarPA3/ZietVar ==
  InZiet : Inport  Orientation=left  Port=1  LatchInput=off
  Constant{,1..2,4} (4 alike) : Constant
  Contrôleur : Stateflow chart  Orientation=left
  Divide{1..4} (4 alike) : Product  Inputs=*/  OutScaling=2^-10
  Rct : Fcn  Expr=u*(3147.77*(1/((1E6*abs(u))^0.7199)))*1000
  Sum : Sum  Inputs=|++
  Sum1 : Sum  Inputs=|++
  Zcpa : Subsystem
  Zw : Subsystem
  OutZiet : Outport  Orientation=left
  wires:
  Constant/1 -> Divide1/1
  Constant1/1 -> Divide2/1
  Constant2/1 -> Divide3/1
  Zcpa/1(OutZcpa) -> Divide3/2
  Zw/1(OutZw) -> Divide2/2
  Rct/1 -> Divide1/2
  Divide3/1 -> Sum/1
  Constant4/1 -> Divide4/1
  Divide2/1 -> Sum/2
  Sum/1 -> Sum1/1
  Divide1/1 -> Sum1/2
  Sum1/1 -> Divide4/2
  Contrôleur/2(temp) -> Rct/1, Zw/1(InZw), Zcpa/1(InZcpa)
  InZiet/1 -> Contrôleur/1(u)
  Contrôleur/1(y) -> OutZiet/1
  Divide4/1 -> Contrôleur/2(calc)

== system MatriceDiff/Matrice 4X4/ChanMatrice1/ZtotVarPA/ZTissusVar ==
  IStim : Inport  Orientation=left  Port=1  LatchInput=off
  Vref : Inport  Port=2  LatchInput=off
  Constant : Constant
  Contrôleur : Stateflow chart  Orientation=left
  Divide : Product  Inputs=*/  OutScaling=2^-10
  Divide1 : Product  Inputs=*/  OutScaling=2^-10
  Divide2 : Product  Inputs=*/  OutScaling=2^-10
  Rext1 : Fcn  Expr=u*(1.6342*((abs(u)*1E6)^0.1267))*1E3
  Sum1 : Sum  Inputs=|++
  ZTissusInt : Subsystem
  Vout : Outport  Orientation=left
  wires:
  Constant/1 -> Divide/1, Divide1/1, Divide2/1
  ZTissusInt/1(Vout) -> Divide/2
  Rext1/1 -> Divide1/2
  Divide/1 -> Sum1/1
  Divide1/1 -> Sum1/2
  Sum1/1 -> Divide2/2
  Vref/1 -> ZTissusInt/2(VRefIn)
  Divide2/1 -> Contrôleur/2(calc)
  Contrôleur/2(temp) -> Rext1/1, ZTissusInt/1(InStim)
  IStim/1 -> Contrôleur/1(u)
  Contrôleur/1(y) -> Vout/1

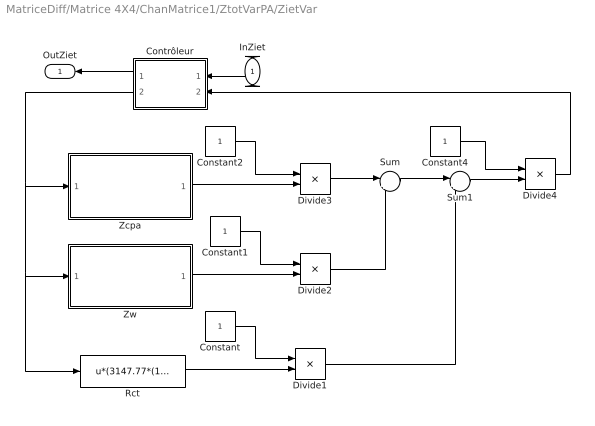
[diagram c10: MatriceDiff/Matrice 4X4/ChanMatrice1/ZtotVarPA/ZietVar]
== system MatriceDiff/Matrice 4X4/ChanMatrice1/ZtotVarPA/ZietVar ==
  InZiet : Inport  Orientation=left  Port=1  LatchInput=off
  Constant{,1..2,4} (4 alike) : Constant
  Contrôleur : Stateflow chart  Orientation=left
  Divide{1..4} (4 alike) : Product  Inputs=*/  OutScaling=2^-10
  Rct : Fcn  Expr=u*(3147.77*(1/((1E6*abs(u))^0.7199)))*1000
  Sum : Sum  Inputs=|++
  Sum1 : Sum  Inputs=|++
  Zcpa : Subsystem
  Zw : Subsystem
  OutZiet : Outport  Orientation=left
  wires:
  Constant/1 -> Divide1/1
  Constant1/1 -> Divide2/1
  Constant2/1 -> Divide3/1
  Zcpa/1(OutZcpa) -> Divide3/2
  Zw/1(OutZw) -> Divide2/2
  Rct/1 -> Divide1/2
  Divide3/1 -> Sum/1
  Constant4/1 -> Divide4/1
  Divide2/1 -> Sum/2
  Sum/1 -> Sum1/1
  Divide1/1 -> Sum1/2
  Sum1/1 -> Divide4/2
  Contrôleur/2(temp) -> Rct/1, Zw/1(InZw), Zcpa/1(InZcpa)
  InZiet/1 -> Contrôleur/1(u)
  Contrôleur/1(y) -> OutZiet/1
  Divide4/1 -> Contrôleur/2(calc)

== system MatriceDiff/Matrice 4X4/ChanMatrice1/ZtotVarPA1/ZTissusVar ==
  IStim : Inport  Orientation=left  Port=1  LatchInput=off
  Vref : Inport  Port=2  LatchInput=off
  Constant : Constant
  Contrôleur : Stateflow chart  Orientation=left
  Divide : Product  Inputs=*/  OutScaling=2^-10
  Divide1 : Product  Inputs=*/  OutScaling=2^-10
  Divide2 : Product  Inputs=*/  OutScaling=2^-10
  Rext1 : Fcn  Expr=u*(1.6342*((abs(u)*1E6)^0.1267))*1E3
  Sum1 : Sum  Inputs=|++
  ZTissusInt : Subsystem
  Vout : Outport  Orientation=left
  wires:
  Constant/1 -> Divide/1, Divide1/1, Divide2/1
  ZTissusInt/1(Vout) -> Divide/2
  Rext1/1 -> Divide1/2
  Divide/1 -> Sum1/1
  Divide1/1 -> Sum1/2
  Sum1/1 -> Divide2/2
  Vref/1 -> ZTissusInt/2(VRefIn)
  Divide2/1 -> Contrôleur/2(calc)
  Contrôleur/2(temp) -> Rext1/1, ZTissusInt/1(InStim)
  IStim/1 -> Contrôleur/1(u)
  Contrôleur/1(y) -> Vout/1

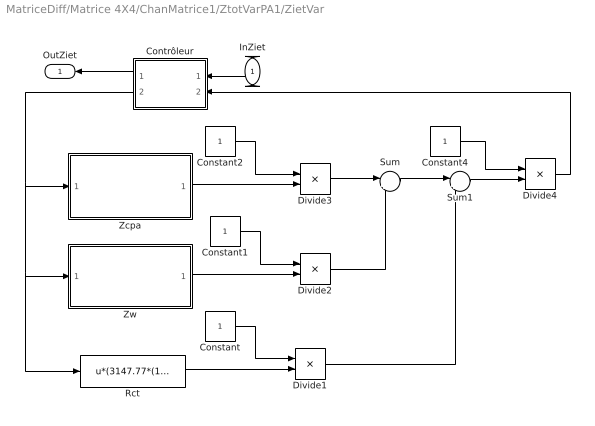
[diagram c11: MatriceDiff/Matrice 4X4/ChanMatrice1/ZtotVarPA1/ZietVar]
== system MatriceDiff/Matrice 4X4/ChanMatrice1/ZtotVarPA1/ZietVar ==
  InZiet : Inport  Orientation=left  Port=1  LatchInput=off
  Constant{,1..2,4} (4 alike) : Constant
  Contrôleur : Stateflow chart  Orientation=left
  Divide{1..4} (4 alike) : Product  Inputs=*/  OutScaling=2^-10
  Rct : Fcn  Expr=u*(3147.77*(1/((1E6*abs(u))^0.7199)))*1000
  Sum : Sum  Inputs=|++
  Sum1 : Sum  Inputs=|++
  Zcpa : Subsystem
  Zw : Subsystem
  OutZiet : Outport  Orientation=left
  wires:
  Constant/1 -> Divide1/1
  Constant1/1 -> Divide2/1
  Constant2/1 -> Divide3/1
  Zcpa/1(OutZcpa) -> Divide3/2
  Zw/1(OutZw) -> Divide2/2
  Rct/1 -> Divide1/2
  Divide3/1 -> Sum/1
  Constant4/1 -> Divide4/1
  Divide2/1 -> Sum/2
  Sum/1 -> Sum1/1
  Divide1/1 -> Sum1/2
  Sum1/1 -> Divide4/2
  Contrôleur/2(temp) -> Rct/1, Zw/1(InZw), Zcpa/1(InZcpa)
  InZiet/1 -> Contrôleur/1(u)
  Contrôleur/1(y) -> OutZiet/1
  Divide4/1 -> Contrôleur/2(calc)

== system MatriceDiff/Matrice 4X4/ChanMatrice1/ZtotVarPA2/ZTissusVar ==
  IStim : Inport  Orientation=left  Port=1  LatchInput=off
  Vref : Inport  Port=2  LatchInput=off
  Constant : Constant
  Contrôleur : Stateflow chart  Orientation=left
  Divide : Product  Inputs=*/  OutScaling=2^-10
  Divide1 : Product  Inputs=*/  OutScaling=2^-10
  Divide2 : Product  Inputs=*/  OutScaling=2^-10
  Rext1 : Fcn  Expr=u*(1.6342*((abs(u)*1E6)^0.1267))*1E3
  Sum1 : Sum  Inputs=|++
  ZTissusInt : Subsystem
  Vout : Outport  Orientation=left
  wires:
  Constant/1 -> Divide/1, Divide1/1, Divide2/1
  ZTissusInt/1(Vout) -> Divide/2
  Rext1/1 -> Divide1/2
  Divide/1 -> Sum1/1
  Divide1/1 -> Sum1/2
  Sum1/1 -> Divide2/2
  Vref/1 -> ZTissusInt/2(VRefIn)
  Divide2/1 -> Contrôleur/2(calc)
  Contrôleur/2(temp) -> Rext1/1, ZTissusInt/1(InStim)
  IStim/1 -> Contrôleur/1(u)
  Contrôleur/1(y) -> Vout/1

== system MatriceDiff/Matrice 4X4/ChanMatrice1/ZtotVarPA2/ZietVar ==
  InZiet : Inport  Orientation=left  Port=1  LatchInput=off
  Constant{,1..2,4} (4 alike) : Constant
  Contrôleur : Stateflow chart  Orientation=left
  Divide{1..4} (4 alike) : Product  Inputs=*/  OutScaling=2^-10
  Rct : Fcn  Expr=u*(3147.77*(1/((1E6*abs(u))^0.7199)))*1000
  Sum : Sum  Inputs=|++
  Sum1 : Sum  Inputs=|++
  Zcpa : Subsystem
  Zw : Subsystem
  OutZiet : Outport  Orientation=left
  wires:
  Constant/1 -> Divide1/1
  Constant1/1 -> Divide2/1
  Constant2/1 -> Divide3/1
  Zcpa/1(OutZcpa) -> Divide3/2
  Zw/1(OutZw) -> Divide2/2
  Rct/1 -> Divide1/2
  Divide3/1 -> Sum/1
  Constant4/1 -> Divide4/1
  Divide2/1 -> Sum/2
  Sum/1 -> Sum1/1
  Divide1/1 -> Sum1/2
  Sum1/1 -> Divide4/2
  Contrôleur/2(temp) -> Rct/1, Zw/1(InZw), Zcpa/1(InZcpa)
  InZiet/1 -> Contrôleur/1(u)
  Contrôleur/1(y) -> OutZiet/1
  Divide4/1 -> Contrôleur/2(calc)

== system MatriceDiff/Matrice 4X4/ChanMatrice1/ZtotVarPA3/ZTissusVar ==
  IStim : Inport  Orientation=left  Port=1  LatchInput=off
  Vref : Inport  Port=2  LatchInput=off
  Constant : Constant
  Contrôleur : Stateflow chart  Orientation=left
  Divide : Product  Inputs=*/  OutScaling=2^-10
  Divide1 : Product  Inputs=*/  OutScaling=2^-10
  Divide2 : Product  Inputs=*/  OutScaling=2^-10
  Rext1 : Fcn  Expr=u*(1.6342*((abs(u)*1E6)^0.1267))*1E3
  Sum1 : Sum  Inputs=|++
  ZTissusInt : Subsystem
  Vout : Outport  Orientation=left
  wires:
  Constant/1 -> Divide/1, Divide1/1, Divide2/1
  ZTissusInt/1(Vout) -> Divide/2
  Rext1/1 -> Divide1/2
  Divide/1 -> Sum1/1
  Divide1/1 -> Sum1/2
  Sum1/1 -> Divide2/2
  Vref/1 -> ZTissusInt/2(VRefIn)
  Divide2/1 -> Contrôleur/2(calc)
  Contrôleur/2(temp) -> Rext1/1, ZTissusInt/1(InStim)
  IStim/1 -> Contrôleur/1(u)
  Contrôleur/1(y) -> Vout/1

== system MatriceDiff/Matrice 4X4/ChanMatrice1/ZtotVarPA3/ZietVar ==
  InZiet : Inport  Orientation=left  Port=1  LatchInput=off
  Constant{,1..2,4} (4 alike) : Constant
  Contrôleur : Stateflow chart  Orientation=left
  Divide{1..4} (4 alike) : Product  Inputs=*/  OutScaling=2^-10
  Rct : Fcn  Expr=u*(3147.77*(1/((1E6*abs(u))^0.7199)))*1000
  Sum : Sum  Inputs=|++
  Sum1 : Sum  Inputs=|++
  Zcpa : Subsystem
  Zw : Subsystem
  OutZiet : Outport  Orientation=left
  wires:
  Constant/1 -> Divide1/1
  Constant1/1 -> Divide2/1
  Constant2/1 -> Divide3/1
  Zcpa/1(OutZcpa) -> Divide3/2
  Zw/1(OutZw) -> Divide2/2
  Rct/1 -> Divide1/2
  Divide3/1 -> Sum/1
  Constant4/1 -> Divide4/1
  Divide2/1 -> Sum/2
  Sum/1 -> Sum1/1
  Divide1/1 -> Sum1/2
  Sum1/1 -> Divide4/2
  Contrôleur/2(temp) -> Rct/1, Zw/1(InZw), Zcpa/1(InZcpa)
  InZiet/1 -> Contrôleur/1(u)
  Contrôleur/1(y) -> OutZiet/1
  Divide4/1 -> Contrôleur/2(calc)

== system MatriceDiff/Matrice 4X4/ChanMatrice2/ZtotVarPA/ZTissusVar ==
  IStim : Inport  Orientation=left  Port=1  LatchInput=off
  Vref : Inport  Port=2  LatchInput=off
  Constant : Constant
  Contrôleur : Stateflow chart  Orientation=left
  Divide : Product  Inputs=*/  OutScaling=2^-10
  Divide1 : Product  Inputs=*/  OutScaling=2^-10
  Divide2 : Product  Inputs=*/  OutScaling=2^-10
  Rext1 : Fcn  Expr=u*(1.6342*((abs(u)*1E6)^0.1267))*1E3
  Sum1 : Sum  Inputs=|++
  ZTissusInt : Subsystem
  Vout : Outport  Orientation=left
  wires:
  Constant/1 -> Divide/1, Divide1/1, Divide2/1
  ZTissusInt/1(Vout) -> Divide/2
  Rext1/1 -> Divide1/2
  Divide/1 -> Sum1/1
  Divide1/1 -> Sum1/2
  Sum1/1 -> Divide2/2
  Vref/1 -> ZTissusInt/2(VRefIn)
  Divide2/1 -> Contrôleur/2(calc)
  Contrôleur/2(temp) -> Rext1/1, ZTissusInt/1(InStim)
  IStim/1 -> Contrôleur/1(u)
  Contrôleur/1(y) -> Vout/1

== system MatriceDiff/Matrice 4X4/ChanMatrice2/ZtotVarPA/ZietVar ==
  InZiet : Inport  Orientation=left  Port=1  LatchInput=off
  Constant{,1..2,4} (4 alike) : Constant
  Contrôleur : Stateflow chart  Orientation=left
  Divide{1..4} (4 alike) : Product  Inputs=*/  OutScaling=2^-10
  Rct : Fcn  Expr=u*(3147.77*(1/((1E6*abs(u))^0.7199)))*1000
  Sum : Sum  Inputs=|++
  Sum1 : Sum  Inputs=|++
  Zcpa : Subsystem
  Zw : Subsystem
  OutZiet : Outport  Orientation=left
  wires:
  Constant/1 -> Divide1/1
  Constant1/1 -> Divide2/1
  Constant2/1 -> Divide3/1
  Zcpa/1(OutZcpa) -> Divide3/2
  Zw/1(OutZw) -> Divide2/2
  Rct/1 -> Divide1/2
  Divide3/1 -> Sum/1
  Constant4/1 -> Divide4/1
  Divide2/1 -> Sum/2
  Sum/1 -> Sum1/1
  Divide1/1 -> Sum1/2
  Sum1/1 -> Divide4/2
  Contrôleur/2(temp) -> Rct/1, Zw/1(InZw), Zcpa/1(InZcpa)
  InZiet/1 -> Contrôleur/1(u)
  Contrôleur/1(y) -> OutZiet/1
  Divide4/1 -> Contrôleur/2(calc)

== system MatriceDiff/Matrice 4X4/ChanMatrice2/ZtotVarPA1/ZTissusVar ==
  IStim : Inport  Orientation=left  Port=1  LatchInput=off
  Vref : Inport  Port=2  LatchInput=off
  Constant : Constant
  Contrôleur : Stateflow chart  Orientation=left
  Divide : Product  Inputs=*/  OutScaling=2^-10
  Divide1 : Product  Inputs=*/  OutScaling=2^-10
  Divide2 : Product  Inputs=*/  OutScaling=2^-10
  Rext1 : Fcn  Expr=u*(1.6342*((abs(u)*1E6)^0.1267))*1E3
  Sum1 : Sum  Inputs=|++
  ZTissusInt : Subsystem
  Vout : Outport  Orientation=left
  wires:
  Constant/1 -> Divide/1, Divide1/1, Divide2/1
  ZTissusInt/1(Vout) -> Divide/2
  Rext1/1 -> Divide1/2
  Divide/1 -> Sum1/1
  Divide1/1 -> Sum1/2
  Sum1/1 -> Divide2/2
  Vref/1 -> ZTissusInt/2(VRefIn)
  Divide2/1 -> Contrôleur/2(calc)
  Contrôleur/2(temp) -> Rext1/1, ZTissusInt/1(InStim)
  IStim/1 -> Contrôleur/1(u)
  Contrôleur/1(y) -> Vout/1

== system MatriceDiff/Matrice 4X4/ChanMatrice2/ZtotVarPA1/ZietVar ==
  InZiet : Inport  Orientation=left  Port=1  LatchInput=off
  Constant{,1..2,4} (4 alike) : Constant
  Contrôleur : Stateflow chart  Orientation=left
  Divide{1..4} (4 alike) : Product  Inputs=*/  OutScaling=2^-10
  Rct : Fcn  Expr=u*(3147.77*(1/((1E6*abs(u))^0.7199)))*1000
  Sum : Sum  Inputs=|++
  Sum1 : Sum  Inputs=|++
  Zcpa : Subsystem
  Zw : Subsystem
  OutZiet : Outport  Orientation=left
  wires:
  Constant/1 -> Divide1/1
  Constant1/1 -> Divide2/1
  Constant2/1 -> Divide3/1
  Zcpa/1(OutZcpa) -> Divide3/2
  Zw/1(OutZw) -> Divide2/2
  Rct/1 -> Divide1/2
  Divide3/1 -> Sum/1
  Constant4/1 -> Divide4/1
  Divide2/1 -> Sum/2
  Sum/1 -> Sum1/1
  Divide1/1 -> Sum1/2
  Sum1/1 -> Divide4/2
  Contrôleur/2(temp) -> Rct/1, Zw/1(InZw), Zcpa/1(InZcpa)
  InZiet/1 -> Contrôleur/1(u)
  Contrôleur/1(y) -> OutZiet/1
  Divide4/1 -> Contrôleur/2(calc)

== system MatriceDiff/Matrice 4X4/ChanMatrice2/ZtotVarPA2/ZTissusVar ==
  IStim : Inport  Orientation=left  Port=1  LatchInput=off
  Vref : Inport  Port=2  LatchInput=off
  Constant : Constant
  Contrôleur : Stateflow chart  Orientation=left
  Divide : Product  Inputs=*/  OutScaling=2^-10
  Divide1 : Product  Inputs=*/  OutScaling=2^-10
  Divide2 : Product  Inputs=*/  OutScaling=2^-10
  Rext1 : Fcn  Expr=u*(1.6342*((abs(u)*1E6)^0.1267))*1E3
  Sum1 : Sum  Inputs=|++
  ZTissusInt : Subsystem
  Vout : Outport  Orientation=left
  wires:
  Constant/1 -> Divide/1, Divide1/1, Divide2/1
  ZTissusInt/1(Vout) -> Divide/2
  Rext1/1 -> Divide1/2
  Divide/1 -> Sum1/1
  Divide1/1 -> Sum1/2
  Sum1/1 -> Divide2/2
  Vref/1 -> ZTissusInt/2(VRefIn)
  Divide2/1 -> Contrôleur/2(calc)
  Contrôleur/2(temp) -> Rext1/1, ZTissusInt/1(InStim)
  IStim/1 -> Contrôleur/1(u)
  Contrôleur/1(y) -> Vout/1

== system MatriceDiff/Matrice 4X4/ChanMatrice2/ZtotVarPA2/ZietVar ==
  InZiet : Inport  Orientation=left  Port=1  LatchInput=off
  Constant{,1..2,4} (4 alike) : Constant
  Contrôleur : Stateflow chart  Orientation=left
  Divide{1..4} (4 alike) : Product  Inputs=*/  OutScaling=2^-10
  Rct : Fcn  Expr=u*(3147.77*(1/((1E6*abs(u))^0.7199)))*1000
  Sum : Sum  Inputs=|++
  Sum1 : Sum  Inputs=|++
  Zcpa : Subsystem
  Zw : Subsystem
  OutZiet : Outport  Orientation=left
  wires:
  Constant/1 -> Divide1/1
  Constant1/1 -> Divide2/1
  Constant2/1 -> Divide3/1
  Zcpa/1(OutZcpa) -> Divide3/2
  Zw/1(OutZw) -> Divide2/2
  Rct/1 -> Divide1/2
  Divide3/1 -> Sum/1
  Constant4/1 -> Divide4/1
  Divide2/1 -> Sum/2
  Sum/1 -> Sum1/1
  Divide1/1 -> Sum1/2
  Sum1/1 -> Divide4/2
  Contrôleur/2(temp) -> Rct/1, Zw/1(InZw), Zcpa/1(InZcpa)
  InZiet/1 -> Contrôleur/1(u)
  Contrôleur/1(y) -> OutZiet/1
  Divide4/1 -> Contrôleur/2(calc)

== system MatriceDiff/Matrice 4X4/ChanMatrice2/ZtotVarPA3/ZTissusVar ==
  IStim : Inport  Orientation=left  Port=1  LatchInput=off
  Vref : Inport  Port=2  LatchInput=off
  Constant : Constant
  Contrôleur : Stateflow chart  Orientation=left
  Divide : Product  Inputs=*/  OutScaling=2^-10
  Divide1 : Product  Inputs=*/  OutScaling=2^-10
  Divide2 : Product  Inputs=*/  OutScaling=2^-10
  Rext1 : Fcn  Expr=u*(1.6342*((abs(u)*1E6)^0.1267))*1E3
  Sum1 : Sum  Inputs=|++
  ZTissusInt : Subsystem
  Vout : Outport  Orientation=left
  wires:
  Constant/1 -> Divide/1, Divide1/1, Divide2/1
  ZTissusInt/1(Vout) -> Divide/2
  Rext1/1 -> Divide1/2
  Divide/1 -> Sum1/1
  Divide1/1 -> Sum1/2
  Sum1/1 -> Divide2/2
  Vref/1 -> ZTissusInt/2(VRefIn)
  Divide2/1 -> Contrôleur/2(calc)
  Contrôleur/2(temp) -> Rext1/1, ZTissusInt/1(InStim)
  IStim/1 -> Contrôleur/1(u)
  Contrôleur/1(y) -> Vout/1

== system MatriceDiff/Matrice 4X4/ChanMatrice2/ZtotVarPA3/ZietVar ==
  InZiet : Inport  Orientation=left  Port=1  LatchInput=off
  Constant{,1..2,4} (4 alike) : Constant
  Contrôleur : Stateflow chart  Orientation=left
  Divide{1..4} (4 alike) : Product  Inputs=*/  OutScaling=2^-10
  Rct : Fcn  Expr=u*(3147.77*(1/((1E6*abs(u))^0.7199)))*1000
  Sum : Sum  Inputs=|++
  Sum1 : Sum  Inputs=|++
  Zcpa : Subsystem
  Zw : Subsystem
  OutZiet : Outport  Orientation=left
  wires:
  Constant/1 -> Divide1/1
  Constant1/1 -> Divide2/1
  Constant2/1 -> Divide3/1
  Zcpa/1(OutZcpa) -> Divide3/2
  Zw/1(OutZw) -> Divide2/2
  Rct/1 -> Divide1/2
  Divide3/1 -> Sum/1
  Constant4/1 -> Divide4/1
  Divide2/1 -> Sum/2
  Sum/1 -> Sum1/1
  Divide1/1 -> Sum1/2
  Sum1/1 -> Divide4/2
  Contrôleur/2(temp) -> Rct/1, Zw/1(InZw), Zcpa/1(InZcpa)
  InZiet/1 -> Contrôleur/1(u)
  Contrôleur/1(y) -> OutZiet/1
  Divide4/1 -> Contrôleur/2(calc)

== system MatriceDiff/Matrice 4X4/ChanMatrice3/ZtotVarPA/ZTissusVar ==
  IStim : Inport  Orientation=left  Port=1  LatchInput=off
  Vref : Inport  Port=2  LatchInput=off
  Constant : Constant
  Contrôleur : Stateflow chart  Orientation=left
  Divide : Product  Inputs=*/  OutScaling=2^-10
  Divide1 : Product  Inputs=*/  OutScaling=2^-10
  Divide2 : Product  Inputs=*/  OutScaling=2^-10
  Rext1 : Fcn  Expr=u*(1.6342*((abs(u)*1E6)^0.1267))*1E3
  Sum1 : Sum  Inputs=|++
  ZTissusInt : Subsystem
  Vout : Outport  Orientation=left
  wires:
  Constant/1 -> Divide/1, Divide1/1, Divide2/1
  ZTissusInt/1(Vout) -> Divide/2
  Rext1/1 -> Divide1/2
  Divide/1 -> Sum1/1
  Divide1/1 -> Sum1/2
  Sum1/1 -> Divide2/2
  Vref/1 -> ZTissusInt/2(VRefIn)
  Divide2/1 -> Contrôleur/2(calc)
  Contrôleur/2(temp) -> Rext1/1, ZTissusInt/1(InStim)
  IStim/1 -> Contrôleur/1(u)
  Contrôleur/1(y) -> Vout/1

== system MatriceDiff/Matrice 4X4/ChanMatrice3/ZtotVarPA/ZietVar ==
  InZiet : Inport  Orientation=left  Port=1  LatchInput=off
  Constant{,1..2,4} (4 alike) : Constant
  Contrôleur : Stateflow chart  Orientation=left
  Divide{1..4} (4 alike) : Product  Inputs=*/  OutScaling=2^-10
  Rct : Fcn  Expr=u*(3147.77*(1/((1E6*abs(u))^0.7199)))*1000
  Sum : Sum  Inputs=|++
  Sum1 : Sum  Inputs=|++
  Zcpa : Subsystem
  Zw : Subsystem
  OutZiet : Outport  Orientation=left
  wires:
  Constant/1 -> Divide1/1
  Constant1/1 -> Divide2/1
  Constant2/1 -> Divide3/1
  Zcpa/1(OutZcpa) -> Divide3/2
  Zw/1(OutZw) -> Divide2/2
  Rct/1 -> Divide1/2
  Divide3/1 -> Sum/1
  Constant4/1 -> Divide4/1
  Divide2/1 -> Sum/2
  Sum/1 -> Sum1/1
  Divide1/1 -> Sum1/2
  Sum1/1 -> Divide4/2
  Contrôleur/2(temp) -> Rct/1, Zw/1(InZw), Zcpa/1(InZcpa)
  InZiet/1 -> Contrôleur/1(u)
  Contrôleur/1(y) -> OutZiet/1
  Divide4/1 -> Contrôleur/2(calc)

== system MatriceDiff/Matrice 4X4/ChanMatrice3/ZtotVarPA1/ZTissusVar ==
  IStim : Inport  Orientation=left  Port=1  LatchInput=off
  Vref : Inport  Port=2  LatchInput=off
  Constant : Constant
  Contrôleur : Stateflow chart  Orientation=left
  Divide : Product  Inputs=*/  OutScaling=2^-10
  Divide1 : Product  Inputs=*/  OutScaling=2^-10
  Divide2 : Product  Inputs=*/  OutScaling=2^-10
  Rext1 : Fcn  Expr=u*(1.6342*((abs(u)*1E6)^0.1267))*1E3
  Sum1 : Sum  Inputs=|++
  ZTissusInt : Subsystem
  Vout : Outport  Orientation=left
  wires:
  Constant/1 -> Divide/1, Divide1/1, Divide2/1
  ZTissusInt/1(Vout) -> Divide/2
  Rext1/1 -> Divide1/2
  Divide/1 -> Sum1/1
  Divide1/1 -> Sum1/2
  Sum1/1 -> Divide2/2
  Vref/1 -> ZTissusInt/2(VRefIn)
  Divide2/1 -> Contrôleur/2(calc)
  Contrôleur/2(temp) -> Rext1/1, ZTissusInt/1(InStim)
  IStim/1 -> Contrôleur/1(u)
  Contrôleur/1(y) -> Vout/1

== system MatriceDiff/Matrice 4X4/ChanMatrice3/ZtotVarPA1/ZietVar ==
  InZiet : Inport  Orientation=left  Port=1  LatchInput=off
  Constant{,1..2,4} (4 alike) : Constant
  Contrôleur : Stateflow chart  Orientation=left
  Divide{1..4} (4 alike) : Product  Inputs=*/  OutScaling=2^-10
  Rct : Fcn  Expr=u*(3147.77*(1/((1E6*abs(u))^0.7199)))*1000
  Sum : Sum  Inputs=|++
  Sum1 : Sum  Inputs=|++
  Zcpa : Subsystem
  Zw : Subsystem
  OutZiet : Outport  Orientation=left
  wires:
  Constant/1 -> Divide1/1
  Constant1/1 -> Divide2/1
  Constant2/1 -> Divide3/1
  Zcpa/1(OutZcpa) -> Divide3/2
  Zw/1(OutZw) -> Divide2/2
  Rct/1 -> Divide1/2
  Divide3/1 -> Sum/1
  Constant4/1 -> Divide4/1
  Divide2/1 -> Sum/2
  Sum/1 -> Sum1/1
  Divide1/1 -> Sum1/2
  Sum1/1 -> Divide4/2
  Contrôleur/2(temp) -> Rct/1, Zw/1(InZw), Zcpa/1(InZcpa)
  InZiet/1 -> Contrôleur/1(u)
  Contrôleur/1(y) -> OutZiet/1
  Divide4/1 -> Contrôleur/2(calc)

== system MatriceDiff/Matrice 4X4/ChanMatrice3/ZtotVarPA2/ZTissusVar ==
  IStim : Inport  Orientation=left  Port=1  LatchInput=off
  Vref : Inport  Port=2  LatchInput=off
  Constant : Constant
  Contrôleur : Stateflow chart  Orientation=left
  Divide : Product  Inputs=*/  OutScaling=2^-10
  Divide1 : Product  Inputs=*/  OutScaling=2^-10
  Divide2 : Product  Inputs=*/  OutScaling=2^-10
  Rext1 : Fcn  Expr=u*(1.6342*((abs(u)*1E6)^0.1267))*1E3
  Sum1 : Sum  Inputs=|++
  ZTissusInt : Subsystem
  Vout : Outport  Orientation=left
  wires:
  Constant/1 -> Divide/1, Divide1/1, Divide2/1
  ZTissusInt/1(Vout) -> Divide/2
  Rext1/1 -> Divide1/2
  Divide/1 -> Sum1/1
  Divide1/1 -> Sum1/2
  Sum1/1 -> Divide2/2
  Vref/1 -> ZTissusInt/2(VRefIn)
  Divide2/1 -> Contrôleur/2(calc)
  Contrôleur/2(temp) -> Rext1/1, ZTissusInt/1(InStim)
  IStim/1 -> Contrôleur/1(u)
  Contrôleur/1(y) -> Vout/1

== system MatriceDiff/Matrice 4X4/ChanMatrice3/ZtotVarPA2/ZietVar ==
  InZiet : Inport  Orientation=left  Port=1  LatchInput=off
  Constant{,1..2,4} (4 alike) : Constant
  Contrôleur : Stateflow chart  Orientation=left
  Divide{1..4} (4 alike) : Product  Inputs=*/  OutScaling=2^-10
  Rct : Fcn  Expr=u*(3147.77*(1/((1E6*abs(u))^0.7199)))*1000
  Sum : Sum  Inputs=|++
  Sum1 : Sum  Inputs=|++
  Zcpa : Subsystem
  Zw : Subsystem
  OutZiet : Outport  Orientation=left
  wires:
  Constant/1 -> Divide1/1
  Constant1/1 -> Divide2/1
  Constant2/1 -> Divide3/1
  Zcpa/1(OutZcpa) -> Divide3/2
  Zw/1(OutZw) -> Divide2/2
  Rct/1 -> Divide1/2
  Divide3/1 -> Sum/1
  Constant4/1 -> Divide4/1
  Divide2/1 -> Sum/2
  Sum/1 -> Sum1/1
  Divide1/1 -> Sum1/2
  Sum1/1 -> Divide4/2
  Contrôleur/2(temp) -> Rct/1, Zw/1(InZw), Zcpa/1(InZcpa)
  InZiet/1 -> Contrôleur/1(u)
  Contrôleur/1(y) -> OutZiet/1
  Divide4/1 -> Contrôleur/2(calc)

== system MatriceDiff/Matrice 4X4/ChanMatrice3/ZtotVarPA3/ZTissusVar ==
  IStim : Inport  Orientation=left  Port=1  LatchInput=off
  Vref : Inport  Port=2  LatchInput=off
  Constant : Constant
  Contrôleur : Stateflow chart  Orientation=left
  Divide : Product  Inputs=*/  OutScaling=2^-10
  Divide1 : Product  Inputs=*/  OutScaling=2^-10
  Divide2 : Product  Inputs=*/  OutScaling=2^-10
  Rext1 : Fcn  Expr=u*(1.6342*((abs(u)*1E6)^0.1267))*1E3
  Sum1 : Sum  Inputs=|++
  ZTissusInt : Subsystem
  Vout : Outport  Orientation=left
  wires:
  Constant/1 -> Divide/1, Divide1/1, Divide2/1
  ZTissusInt/1(Vout) -> Divide/2
  Rext1/1 -> Divide1/2
  Divide/1 -> Sum1/1
  Divide1/1 -> Sum1/2
  Sum1/1 -> Divide2/2
  Vref/1 -> ZTissusInt/2(VRefIn)
  Divide2/1 -> Contrôleur/2(calc)
  Contrôleur/2(temp) -> Rext1/1, ZTissusInt/1(InStim)
  IStim/1 -> Contrôleur/1(u)
  Contrôleur/1(y) -> Vout/1

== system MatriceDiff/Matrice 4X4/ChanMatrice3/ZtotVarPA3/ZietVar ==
  InZiet : Inport  Orientation=left  Port=1  LatchInput=off
  Constant{,1..2,4} (4 alike) : Constant
  Contrôleur : Stateflow chart  Orientation=left
  Divide{1..4} (4 alike) : Product  Inputs=*/  OutScaling=2^-10
  Rct : Fcn  Expr=u*(3147.77*(1/((1E6*abs(u))^0.7199)))*1000
  Sum : Sum  Inputs=|++
  Sum1 : Sum  Inputs=|++
  Zcpa : Subsystem
  Zw : Subsystem
  OutZiet : Outport  Orientation=left
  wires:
  Constant/1 -> Divide1/1
  Constant1/1 -> Divide2/1
  Constant2/1 -> Divide3/1
  Zcpa/1(OutZcpa) -> Divide3/2
  Zw/1(OutZw) -> Divide2/2
  Rct/1 -> Divide1/2
  Divide3/1 -> Sum/1
  Constant4/1 -> Divide4/1
  Divide2/1 -> Sum/2
  Sum/1 -> Sum1/1
  Divide1/1 -> Sum1/2
  Sum1/1 -> Divide4/2
  Contrôleur/2(temp) -> Rct/1, Zw/1(InZw), Zcpa/1(InZcpa)
  InZiet/1 -> Contrôleur/1(u)
  Contrôleur/1(y) -> OutZiet/1
  Divide4/1 -> Contrôleur/2(calc)
